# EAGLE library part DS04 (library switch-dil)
DIL/CODE SWITCH
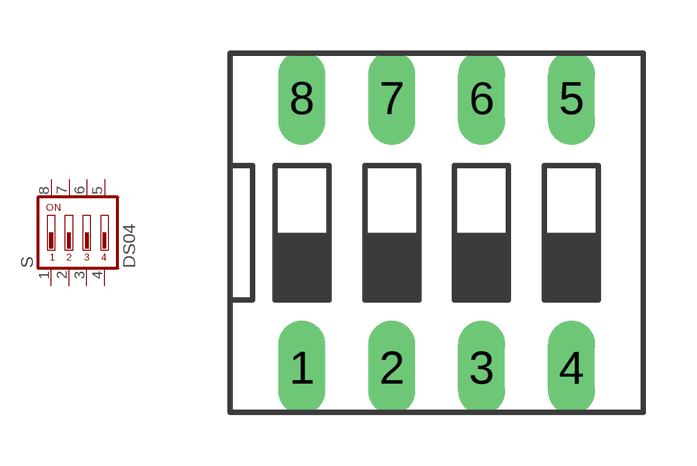
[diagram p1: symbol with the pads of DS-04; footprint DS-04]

Designator prefix S

## DS04 (OC_FARNELL: 9471570; OC_NEWARK: unknown)  [DS-04]
1  1  pas
2  2  pas
3  3  pas
4  4  pas
5  5  pas
6  6  pas
7  7  pas
8  8  pas

## Footprint DS-04 (pad centres in mm)
DIL/CODE SWITCH Mors distributor Buerklin, 17G554
drill 0.813 long: 1 -3.81,-3.81; 2 -1.27,-3.81; 3 1.27,-3.81; 4 3.81,-3.81; 5 3.81,3.81; 6 1.27,3.81; 7 -1.27,3.81; 8 -3.81,3.81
